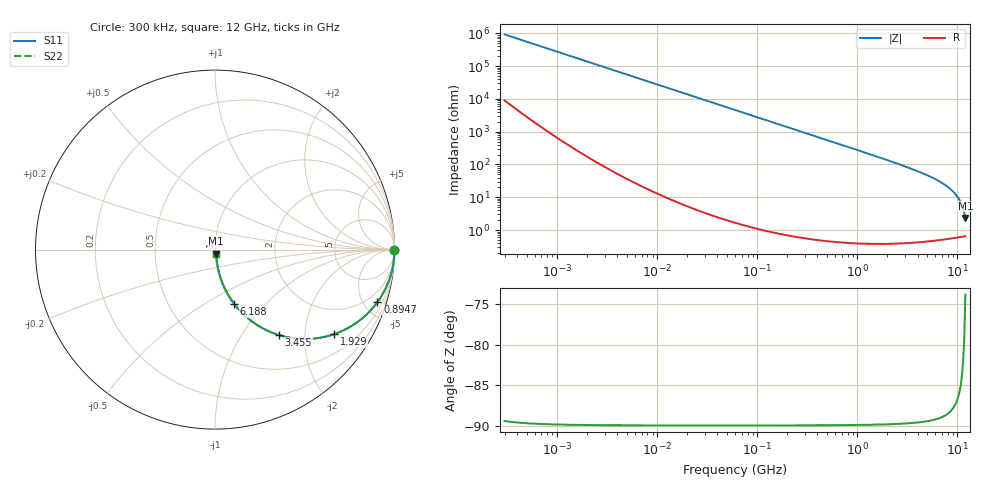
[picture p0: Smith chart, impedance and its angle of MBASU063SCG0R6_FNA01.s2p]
! MBASU063SCG0R6_FNA01  S-PARAMETER MODEL  ( Standard Model )
! Model Generated by TAIYO YUDEN Corporation (http://www.ty-top.com)
! Version 1.0
! TAIYO YUDEN Control No. 230609
! Copyright(c) 2023 TAIYO YUDEN CO.,LTD. All Rights Reserved.
! Product Description (link to TY-COMPAS)
! https://ds.yuden.co.jp/TYCOMPAS/or/detail?pn=MBASU063SCG0R6BFNA01&u=M
! Products Name : Multilayer Ceramic Capacitors
! Characteristics :
!  Capacitance : 0.6 [pF] , Rated Voltage : 50 [V] , TCC : CG / C0G
!  Case Size : 0.6 x 0.3 / 0.024 x 0.012 [mm/inch] , Thickness : 0.3 / 0.012 [mm/inch]
!  (Conditions: Temperature = 25 [degC] , DC Bias Voltage = 0 [V])
! External Node Assignments :
!  1  o---| |---o  2
! GND o---------o GND
! Frequency Range : 0.3MHz  -  12000MHz  [ 401 STEP ]
# MHZ S RI R 50
! Freq[MHz].  S11 Real  S11 Imag  S21 Real  S21 Imag  S12 Real  S12 Imag  S22 Real  S22 Imag
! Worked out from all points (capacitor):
!   401 points, 300 kHz to 12 GHz, reference 50 ohm
!   read as one part in series: C = 574 fF near 316.3 kHz
!   lowest |Z| = 2.32 ohm at 12 GHz (marker M1)
!   S11 on the Smith chart (normalised r, x): 300 kHz: open; 894.7 MHz: 1.01, -6.16; 1.929 GHz: 1.01, -2.81; 3.455 GHz: 1.01, -1.48; 6.188 GHz: 1.01, -0.68; 12 GHz: 1.01, -0.04
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0.3  1 -0.000108  1.07e-06 0.000108  1.07e-06 0.000108  1 -0.000108
1.769972  1 -0.000639  1.29e-06 0.000639  1.29e-06 0.000639  1 -0.000639
10.44266  1 -0.00377  1.59e-05 0.00377  1.59e-05 0.00377  1 -0.00377
60  0.9995 -0.0216  0.000476 0.0216  0.000476 0.0216  0.9995 -0.0216
164.1901  0.9965 -0.059  0.00353 0.059  0.00353 0.059  0.9965 -0.059
353.9943  0.9838 -0.1257  0.0162 0.1257  0.0162 0.1257  0.9838 -0.1257
601.3112  0.9547 -0.2075  0.0453 0.2075  0.0453 0.2075  0.9547 -0.2075
894.6982  0.9045 -0.2933  0.0955 0.2933  0.0955 0.2933  0.9045 -0.2933
1331.232  0.8087 -0.3924  0.1913 0.3924  0.1913 0.3924  0.8087 -0.3924
1928.972  0.6628 -0.4714  0.3372 0.4714  0.3372 0.4714  0.6628 -0.4714
2088.533  0.6246 -0.4828  0.3754 0.4828  0.3754 0.4828  0.6246 -0.4828
2722.03  0.4853 -0.4978  0.5147 0.4978  0.5147 0.4978  0.4853 -0.4978
3454.93  0.3559 -0.4761  0.6441 0.4761  0.6441 0.4761  0.3559 -0.4761
4747.894  0.2029 -0.3978  0.7971 0.3978  0.7971 0.3978  0.2029 -0.3978
6188.031  0.1072 -0.3024  0.8928 0.3024  0.8928 0.3024  0.1072 -0.3024
7854.144  0.0493 -0.2046  0.9507 0.2046  0.9507 0.2046  0.0493 -0.2046
8732.115  0.0317 -0.1594  0.9683 0.1594  0.9683 0.1594  0.0317 -0.1594
9454.42  0.0217 -0.1252  0.9783 0.1252  0.9783 0.1252  0.0217 -0.1252
10236.47  0.0143 -0.0909  0.9857 0.0909  0.9857 0.0909  0.0143 -0.0909
10793.46  0.0108 -0.0679  0.9892 0.0679  0.9892 0.0679  0.0108 -0.0679
11686.27  0.00748 -0.0335  0.9925 0.0335  0.9925 0.0335  0.00748 -0.0335
12000  0.00693 -0.022  0.9931 0.022  0.9931 0.022  0.00693 -0.022
